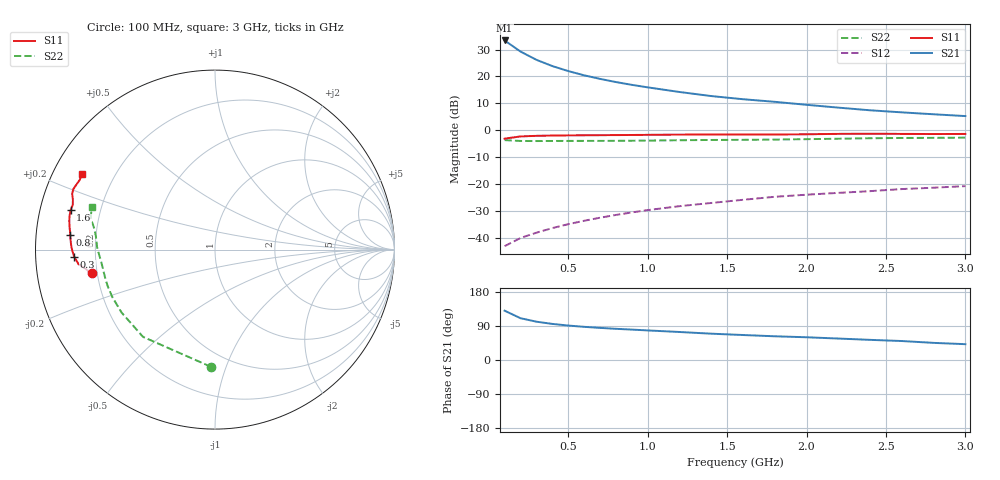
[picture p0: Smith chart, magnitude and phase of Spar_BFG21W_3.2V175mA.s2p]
! Filename: 3_2175bfg21.001
! Title: BFG21W
! Bias: Vce=3.2V; Ic=175mA
! Company: NXP Semiconductors NL
! User: Quality&Reliability T&D
! Measure time: 10 Nov 1999 / 11:43:32
#  MHz  S  MA  R 50
! Freq  S11  S21  S12  S22  :
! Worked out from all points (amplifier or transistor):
!   20 points, 100 MHz to 3 GHz, reference 50 ohm
!   highest |S21| = 33.4 dB at 100 MHz (marker M1)
!   |S21| within 3 dB of that: start of sweep to 172.6 MHz
!   unconditionally stable (mu >= 1): 548.6 MHz to end of sweep
!   at 400 MHz: K = 0.95, MSG = 30.2 dB, |S12| = -36.5 dB
!   at 1.2 GHz: K = 1.06, MAG = 19.8 dB, |S12| = -28.3 dB
!   at 3 GHz: K = 1.05, MAG = 11.7 dB, |S12| = -20.8 dB
!   S11 on the Smith chart (normalised r, x): 100 MHz: 0.18, -0.09; 300 MHz: 0.12, -0.02; 800 MHz: 0.10, +0.05; 1.6 GHz: 0.09, +0.13; 3 GHz: 0.09, +0.26
100  0.6961 -169.0  46.84 130.1  0.006931 60.3  0.6532 -92.0
200  0.7648 -173.9  29.1 110.3  0.009842 58.3  0.6302 -129.5
300  0.7852 -177.1  20.44 101.1  0.01234 62.1  0.6276 -146.0
400  0.7944 -179.4  15.63 95.3  0.01504 65.5  0.6301 -155.0
500  0.8006 178.8  12.62 90.9  0.01777 67.9  0.6314 -160.8
600  0.8042 177.1  10.52 87.5  0.02056 69.7  0.632 -164.9
700  0.8076 175.6  9.029 84.8  0.02347 71.2  0.6323 -168.1
800  0.8105 174.1  7.881 82.3  0.02642 72.3  0.6337 -170.8
900  0.8145 172.7  6.988 80.3  0.02943 73.3  0.6368 -173.2
1000  0.8192 171.4  6.275 78.1  0.03252 73.9  0.6405 -175.3
1200  0.8272 169.0  5.147 73.9  0.03846 74.3  0.6498 -178.7
1400  0.8319 167.0  4.321 69.5  0.04415 74.1  0.6577 178.6
1600  0.8336 164.8  3.772 65.9  0.05059 74.0  0.6614 176.0
1800  0.8309 162.4  3.376 62.6  0.05755 73.7  0.669 173.3
2000  0.8395 160.6  2.97 60.0  0.06296 73.9  0.6804 170.6
2200  0.8543 158.7  2.631 56.6  0.06807 73.5  0.6941 168.4
2400  0.8583 156.9  2.347 53.2  0.07331 72.5  0.7076 166.7
2600  0.8537 155.1  2.148 50.1  0.08014 71.2  0.7165 165.2
2800  0.848 152.8  1.978 45.2  0.08501 69.4  0.7199 163.2
3000  0.8519 150.3  1.831 41.8  0.09094 68.3  0.7265 160.8
